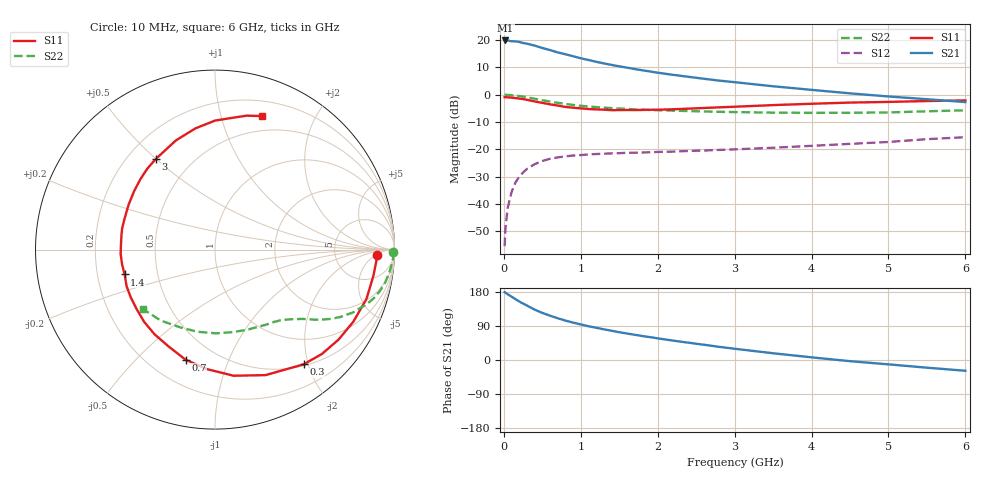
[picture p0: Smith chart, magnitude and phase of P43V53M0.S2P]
! SIEMENS Small Signal Semiconductors
! BFP182
! Si NPN RF Bipolar Junction Transistor in SOT143
! VCE = 3.5 V  IC = 3 mA
! Common Emitter S-Parameters:  March  1996
# GHz  S  MA  R  50
!  f  S11  S21  S12  S22
! GHz  MAG  ANG  MAG  ANG  MAG  ANG  MAG  ANG
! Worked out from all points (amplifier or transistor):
!   36 points, 10 MHz to 6 GHz, reference 50 ohm
!   highest |S21| = 19.9 dB at 20 MHz (marker M1)
!   |S21| within 3 dB of that: start of sweep to 532.7 MHz
!   unconditionally stable (mu >= 1): 1.938 GHz to 5.699 GHz
!   at 250 MHz: K = 0.16, MSG = 23.7 dB, |S12| = -28.5 dB
!   at 1.4 GHz: K = 0.78, MSG = 16.2 dB, |S12| = -21.5 dB
!   at 6 GHz: K = 0.96, MSG = 6.4 dB, |S12| = -15.5 dB
!   S11 on the Smith chart (normalised r, x): 10 MHz: 18, -6; 300 MHz: 0.52, -1.92; 700 MHz: 0.34, -0.71; 1.4 GHz: 0.32, -0.12; 3 GHz: 0.31, +0.50; 6 GHz: 0.34, +1.35
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0.01  0.9031 -1.9  9.662 178.9  0.0017 82.9  0.9944 -0.7
0.02  0.9018 -3.7  9.834 177.9  0.0035 80.0  0.9964 -1.5
0.05  0.8946 -9.3  9.8 173.5  0.0085 87.2  0.9912 -3.7
0.1  0.8876 -18.1  9.514 167.2  0.0165 78.4  0.9804 -7.3
0.15  0.869 -27.6  9.453 160.7  0.0247 74.2  0.9665 -10.8
0.2  0.8516 -36.1  9.24 154.5  0.0317 70.4  0.9471 -14.1
0.25  0.8324 -44.3  8.832 148.9  0.0378 65.4  0.9248 -17.1
0.3  0.8079 -52.3  8.595 143.7  0.044 61.7  0.8981 -19.8
0.4  0.7538 -68.1  7.937 133.0  0.0537 54.3  0.8444 -24.5
0.5  0.7104 -81.6  7.165 124.3  0.0614 47.8  0.7937 -28.2
0.6  0.6675 -93.8  6.562 117.0  0.0675 43.3  0.7519 -30.9
0.7  0.6348 -105.0  5.942 110.2  0.0715 39.3  0.7121 -33.2
0.9  0.5797 -125.5  5.063 98.7  0.0774 33.6  0.6504 -36.6
1.1  0.5481 -142.8  4.321 89.1  0.081 29.3  0.6098 -39.3
1.4  0.5222 -164.6  3.513 77.2  0.0846 25.5  0.5702 -42.9
1.8  0.5271 171.5  2.803 63.3  0.0879 23.5  0.5331 -47.8
2.2  0.5425 152.5  2.313 51.1  0.0911 22.6  0.512 -53.6
3  0.6032 123.1  1.697 29.7  0.1003 22.5  0.4821 -67.6
3.5  0.6462 109.7  1.428 17.8  0.1074 22.4  0.4702 -77.8
4.5  0.7187 90.0  1.06 -3.1  0.1264 21.2  0.4678 -101.9
5.5  0.7668 76.7  0.828 -20.3  0.1541 18.6  0.4977 -127.4
6  0.7883 70.7  0.734 -28.4  0.1672 14.9  0.5194 -140.1
